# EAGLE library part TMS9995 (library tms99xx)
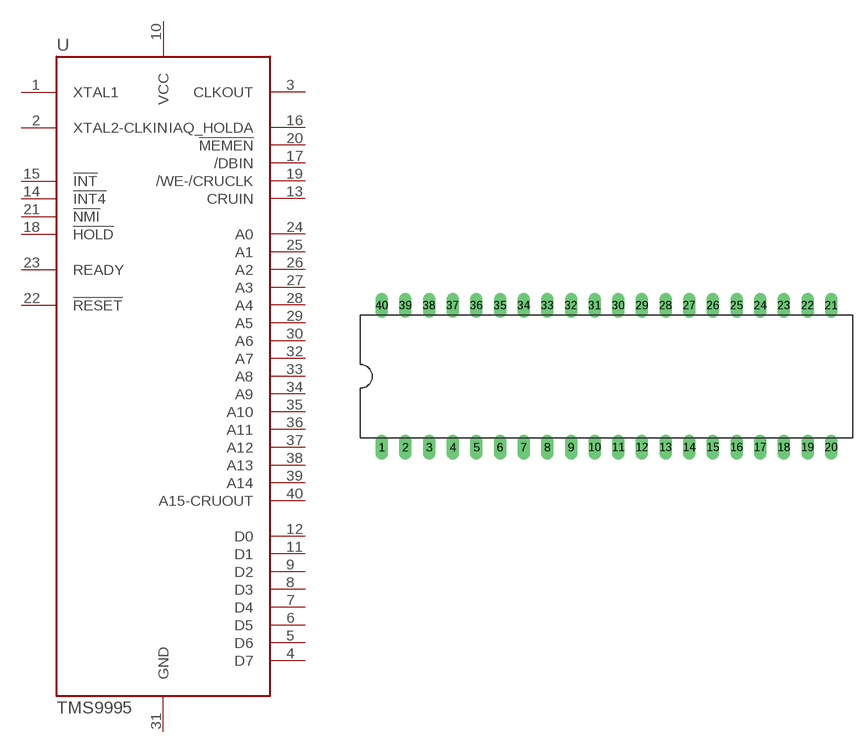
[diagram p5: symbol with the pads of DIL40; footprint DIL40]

Designator prefix -

## TMS9995  [DIL40]
1  XTAL1  in
2  XTAL2-CLKIN  in
3  CLKOUT  out
4  D7
5  D6
6  D5
7  D4
8  D3
9  D2
10  VCC  pwr
11  D1
12  D0
13  CRUIN  in
14  !INT4  in
15  !INT  in
16  IAQ_HOLDA  out
17  /DBIN  out
18  !HOLD  in
19  /WE-/CRUCLK  out
20  !MEMEN  out
21  !NMI  in
22  !RESET  in
23  READY  in
24  A0  out
25  A1  out
26  A2  out
27  A3  out
28  A4  out
29  A5  out
30  A6  out
31  GND  pwr
32  A7  out
33  A8  out
34  A9  out
35  A10  out
36  A11  out
37  A12  out
38  A13  out
39  A14  out
40  A15-CRUOUT  out

## Footprint DIL40 (pad centres in mm)
Dual In Line
drill 0.813 long: 1 -24.13,-7.62; 2 -21.59,-7.62; 3 -19.05,-7.62; 4 -16.51,-7.62; 5 -13.97,-7.62; 6 -11.43,-7.62; 7 -8.89,-7.62; 8 -6.35,-7.62; 9 -3.81,-7.62; 10 -1.27,-7.62; 11 1.27,-7.62; 12 3.81,-7.62; 13 6.35,-7.62; 14 8.89,-7.62; 15 11.43,-7.62; 16 13.97,-7.62; 17 16.51,-7.62; 18 19.05,-7.62; 19 21.59,-7.62; 20 24.13,-7.62; 21 24.13,7.62; 22 21.59,7.62; 23 19.05,7.62; 24 16.51,7.62; 25 13.97,7.62; 26 11.43,7.62; 27 8.89,7.62; 28 6.35,7.62; 29 3.81,7.62; 30 1.27,7.62; 31 -1.27,7.62; 32 -3.81,7.62; 33 -6.35,7.62; 34 -8.89,7.62; 35 -11.43,7.62; 36 -13.97,7.62; 37 -16.51,7.62; 38 -19.05,7.62; 39 -21.59,7.62; 40 -24.13,7.62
